| IBIS file stm32h523_533_lqfp64.ibs
[IBIS ver] 4.2
[File name] stm32h523_533_lqfp64.ibs
[File Rev] 0.2
[Date] 07-05-2024
[Source] Data Created at STMicroelectronics
[Notes]  File originated from ELDO simulations.
[Disclaimer]  This information is for modeling purpose only and is
   not guaranteed. The information is subject to change without
   notice.
[Copyright] Copyright 2024 STMicroelectronics Inc.
|   Component stm32h523_533_lqfp64
[Component] stm32h523_533_lqfp64
[Manufacturer] STMicroelectronics
[Package]
| variable   typ   min   max
R_pkg  0  NA  NA
L_pkg  0  NA  NA
C_pkg  0  NA  NA
[Pin]   signal_name   model_name
1  VBAT  power
2  PC13  io8_ft_i3c_spi_v33
3  PC14-OSC32_IN  io_ft_tamp
4  PC15-OSC32_OUT  io_ft_tamp
5  PH0-OSC_IN  io8_ft_i3c_spi
6  PH1-OSC_OUT  io8_ft_i3c_spi
7  NRST  ioreset_ft_v33
8  PC0  io8_ft_spi
9  PC1  io8_ft_spi
10  PC2  io8_ft_spi
11  PC3  io8_ft_spi
12  VSSA  nc
13  VDDA  nc
14  PA0  io8_ft_spi
15  PA1  io8_ft_spi_tamp
16  PA2  io8_ft_spi
17  PA3  io8_ft_spi
18  VSS  gnd
19  VDD  power
20  PA4  io8_ft_spi
21  PA5  io8_ft_spi
22  PA6  io8_ft_spi
23  PA7  io8_ft_spi
24  PC4  io8_ft_spi
25  PC5  io8_ft_spi
26  PB0  io8_ft_spi
27  PB1  io8_ft_spi
28  PB2  io8_ft_i3c_spi
29  PB10  io8_ft_i3c_spi
30  VCAP  nc
31  VSS  gnd
32  VDD  power
33  PB12  io8_ft_i3c_spi
34  PB13  nc
35  PB14  nc
36  PB15  io8_ft_spi
37  PC6  io8_ft_i3c_spi
38  PC7  io8_ft_i3c_spi
39  PC8  io8_ft_i3c_spi
40  PC9  io8_ft_i3c_spi
41  PA8  io8_ft_i3c_spi
42  PA9  io8_ft_i3c_spi
43  PA10  io8_ft_i3c_spi
44  PA11  io8usb_ft_i3c_spi_phy
45  PA12  io8usb_ft_i3c_spi_phy
46  PA13  io8_ft_i3c_spi
47  VSS  gnd
48  VDD  power
49  PA14  io8_ft_i3c_spi
50  PA15  io8_ft_i3c_spi
51  PC10  io8_ft_i3c_spi
52  PC11  io8_ft_i3c_spi
53  PC12  io8_ft_i3c_spi
54  PD2  io8_ft_i3c_spi
55  PB3  io8_ft_i3c_spi
56  PB4  io8_ft_i3c_spi
57  PB5  io8_ft_i3c_spi
58  PB6  io8_ft_i3c_spi
59  PB7  io8_ft_i3c_spi
60  BOOT0  vpphv
61  PB8  io8_ft_i3c_spi
62  VCAP  nc
63  VSS  gnd
64  VDD  power
[Package Model]   478-lqfp-7x7-64-240319
[Pin Mapping]   pulldown_ref   pullup_ref   | Comment
1  nc  vsw
2  gndio  vddio  | Depending on IO usage
| 2  gndio  vsw  | Depending on IO usage
3  gndio  vddio  | Depending on IO usage
| 3  gndio  vsw  | Depending on IO usage
4  gndio  vddio  | Depending on IO usage
| 4  gndio  vsw  | Depending on IO usage
5  gndio  vddio
6  gndio  vddio
7  gndio  vddio
8  gndio  vddio
9  gndio  vddio
10  gndio  vddio
11  gndio  vddio
12  nc  nc
13  nc  nc
14  gndio  vddio
15  gndio  vddio
16  gndio  vddio
17  gndio  vddio
18  gndio  nc
19  nc  vddio
20  gndio  vddio
21  gndio  vddio
22  gndio  vddio
23  gndio  vddio
24  gndio  vddio
25  gndio  vddio
26  gndio  vddio
27  gndio  vddio
28  gndio  vddio
29  gndio  vddio
30  nc  nc
31  gndio  nc
32  nc  vddio
33  gndio  vddio
34  nc  nc
35  nc  nc
36  gndio  vddio
37  gndio  vddio
38  gndio  vddio
39  gndio  vddio
40  gndio  vddio
41  gndio  vddio
42  gndio  vddio
43  gndio  vddio
44  gndio  vddio
45  gndio  vddio
46  gndio  vddio
47  gndio  nc
48  nc  vddio
49  gndio  vddio
50  gndio  vddio
51  gndio  vddio
52  gndio  vddio
53  gndio  vddio
54  gndio  vddio
55  gndio  vddio
56  gndio  vddio
57  gndio  vddio
58  gndio  vddio
59  gndio  vddio
60  gndio  vddio
61  gndio  vddio
62  nc  nc
63  gndio  nc
64  nc  vddio
|[Diff Pin]  inv_pin  vdiff  tdelay_typ  tdelay_min  tdelay_max
|45  44  NA  NA  NA  NA
[Model Selector] io8_ft_i3c_spi
io8_ft_spi_ls_1v2 "GPIO SPI - 5V tolerant - low speed - 1.2V range"
io8_ft_spi_ls_1v8 "GPIO SPI - 5V tolerant - low speed - 1.8V range"
io8_ft_spi_ls_3v3 "GPIO SPI - 5V tolerant - low speed - 3.3V range"
io8_ft_spi_ms_1v2 "GPIO SPI - 5V tolerant - med speed - 1.2V range"
io8_ft_spi_ms_1v8 "GPIO SPI - 5V tolerant - med speed - 1.8V range"
io8_ft_spi_ms_3v3 "GPIO SPI - 5V tolerant - med speed - 3.3V range"
io8_ft_spi_fs_1v2 "GPIO SPI - 5V tolerant - fast speed - 1.2V range"
io8_ft_spi_fs_1v8 "GPIO SPI - 5V tolerant - fast speed - 1.8V range"
io8_ft_spi_fs_3v3 "GPIO SPI - 5V tolerant - fast speed - 3.3V range"
io8_ft_spi_hs_1v2 "GPIO SPI - 5V tolerant - high speed - 1.2V range"
io8_ft_spi_hs_1v8 "GPIO SPI - 5V tolerant - high speed - 1.8V range"
io8_ft_spi_hs_3v3 "GPIO SPI - 5V tolerant - high speed - 3.3V range"
io8_ft_hslv_spi_ls_1v2 "GPIO SPI low volt opt - 5V tolerant - low speed - 1.2V range"
io8_ft_hslv_spi_ls_1v8 "GPIO SPI low volt opt - 5V tolerant - low speed - 1.8V range"
io8_ft_hslv_spi_ls_2v5 "GPIO SPI low volt opt - 5V tolerant - low speed - 2.5V range"
io8_ft_hslv_spi_ms_1v2 "GPIO SPI low volt opt - 5V tolerant - med speed - 1.2V range"
io8_ft_hslv_spi_ms_1v8 "GPIO SPI low volt opt - 5V tolerant - med speed - 1.8V range"
io8_ft_hslv_spi_ms_2v5 "GPIO SPI low volt opt - 5V tolerant - med speed - 2.5V range"
io8_ft_hslv_spi_fs_1v2 "GPIO SPI low volt opt - 5V tolerant - fast speed - 1.2V range"
io8_ft_hslv_spi_fs_1v8 "GPIO SPI low volt opt - 5V tolerant - fast speed - 1.8V range"
io8_ft_hslv_spi_fs_2v5 "GPIO SPI low volt opt - 5V tolerant - fast speed - 2.5V range"
io8_ft_hslv_spi_hs_1v2 "GPIO SPI low volt opt - 5V tolerant - high speed - 1.2V range"
io8_ft_hslv_spi_hs_1v8 "GPIO SPI low volt opt - 5V tolerant - high speed - 1.8V range"
io8_ft_hslv_spi_hs_2v5 "GPIO SPI low volt opt - 5V tolerant - high speed - 2.5V range"
io8_ft_i3c_spi_ls_1v2 "GPIO SPI with I3C open-drain - 5V tolerant - low speed - 1.2V range"
io8_ft_i3c_spi_ls_1v8 "GPIO SPI with I3C open-drain - 5V tolerant - low speed - 1.8V range"
io8_ft_i3c_spi_ls_3v3 "GPIO SPI with I3C open-drain - 5V tolerant - low speed - 3.3V range"
io8_ft_i3c_spi_ms_1v2 "GPIO SPI with I3C open-drain - 5V tolerant - med speed - 1.2V range"
io8_ft_i3c_spi_ms_1v8 "GPIO SPI with I3C open-drain - 5V tolerant - med speed - 1.8V range"
io8_ft_i3c_spi_ms_3v3 "GPIO SPI with I3C open-drain - 5V tolerant - med speed - 3.3V range"
io8_ft_i3c_spi_fs_1v2 "GPIO SPI with I3C open-drain - 5V tolerant - fast speed - 1.2V range"
io8_ft_i3c_spi_fs_1v8 "GPIO SPI with I3C open-drain - 5V tolerant - fast speed - 1.8V range"
io8_ft_i3c_spi_fs_3v3 "GPIO SPI with I3C open-drain - 5V tolerant - fast speed - 3.3V range"
io8_ft_i3c_spi_hs_1v2 "GPIO SPI with I3C open-drain - 5V tolerant - high speed - 1.2V range"
io8_ft_i3c_spi_hs_1v8 "GPIO SPI with I3C open-drain - 5V tolerant - high speed - 1.8V range"
io8_ft_i3c_spi_hs_3v3 "GPIO SPI with I3C open-drain - 5V tolerant - high speed - 3.3V range"
io8_ft_hslv_i3c_spi_ls_1v2 "GPIO SPI low volt opt with I3C open-drain - 5V tolerant - low speed - 1.2V range"
io8_ft_hslv_i3c_spi_ls_1v8 "GPIO SPI low volt opt with I3C open-drain - 5V tolerant - low speed - 1.8V range"
io8_ft_hslv_i3c_spi_ls_2v5 "GPIO SPI low volt opt with I3C open-drain - 5V tolerant - low speed - 2.5V range"
io8_ft_hslv_i3c_spi_ms_1v2 "GPIO SPI low volt opt with I3C open-drain - 5V tolerant - med speed - 1.2V range"
io8_ft_hslv_i3c_spi_ms_1v8 "GPIO SPI low volt opt with I3C open-drain - 5V tolerant - med speed - 1.8V range"
io8_ft_hslv_i3c_spi_ms_2v5 "GPIO SPI low volt opt with I3C open-drain - 5V tolerant - med speed - 2.5V range"
io8_ft_hslv_i3c_spi_fs_1v2 "GPIO SPI low volt opt with I3C open-drain - 5V tolerant - fast speed - 1.2V range"
io8_ft_hslv_i3c_spi_fs_1v8 "GPIO SPI low volt opt with I3C open-drain - 5V tolerant - fast speed - 1.8V range"
io8_ft_hslv_i3c_spi_fs_2v5 "GPIO SPI low volt opt with I3C open-drain - 5V tolerant - fast speed - 2.5V range"
io8_ft_hslv_i3c_spi_hs_1v2 "GPIO SPI low volt opt with I3C open-drain - 5V tolerant - high speed - 1.2V range"
io8_ft_hslv_i3c_spi_hs_1v8 "GPIO SPI low volt opt with I3C open-drain - 5V tolerant - high speed - 1.8V range"
io8_ft_hslv_i3c_spi_hs_2v5 "GPIO SPI low volt opt with I3C open-drain - 5V tolerant - high speed - 2.5V range"
io8_ft_i3c_fmp_spi_3v3 "GPIO SPI with I3C fm+ open-drain - 5V tolerant - 3.3V range"
io8_ft_i3c_fmp_spi_1v8 "GPIO SPI with I3C fm+ open-drain - 5V tolerant - 1.8V range"
io8_ft_i3c_fmp_spi_1v2 "GPIO SPI with I3C fm+ open-drain - 5V tolerant - 1.2V range"
[Model Selector] io8_ft_i3c_spi_v33
io8_ft_spi_v33_ls_1v2 ""GPIO SPI V33 - 5V tolerant - low speed - 1.2V range"
io8_ft_spi_v33_ls_1v8 ""GPIO SPI V33 - 5V tolerant - low speed - 1.8V range"
io8_ft_spi_v33_ls_3v3 ""GPIO SPI V33 - 5V tolerant - low speed - 3.3V range"
io8_ft_spi_v33_ms_1v2 ""GPIO SPI V33 - 5V tolerant - med speed - 1.2V range"
io8_ft_spi_v33_ms_1v8 ""GPIO SPI V33 - 5V tolerant - med speed - 1.8V range"
io8_ft_spi_v33_ms_3v3 ""GPIO SPI V33 - 5V tolerant - med speed - 3.3V range"
io8_ft_spi_v33_fs_1v2 ""GPIO SPI V33 - 5V tolerant - fast speed - 1.2V range
io8_ft_spi_v33_fs_1v8 ""GPIO SPI V33 - 5V tolerant - fast speed - 1.8V range
io8_ft_spi_v33_fs_3v3 ""GPIO SPI V33 - 5V tolerant - fast speed - 3.3V range
io8_ft_spi_v33_hs_1v2 ""GPIO SPI V33 - 5V tolerant - high speed - 1.2V range
io8_ft_spi_v33_hs_1v8 ""GPIO SPI V33 - 5V tolerant - high speed - 1.8V range
io8_ft_spi_v33_hs_3v3 ""GPIO SPI V33 - 5V tolerant - high speed - 3.3V range
io8_ft_hslv_spi_v33_ls_1v2 "GPIO SPI V33 low volt opt - 5V tolerant - low speed - 1.2V range""
io8_ft_hslv_spi_v33_ls_1v8 "GPIO SPI V33 low volt opt - 5V tolerant - low speed - 1.8V range""
io8_ft_hslv_spi_v33_ls_2v5 "GPIO SPI V33 low volt opt - 5V tolerant - low speed - 2.5V range""
io8_ft_hslv_spi_v33_ms_1v2 "GPIO SPI V33 low volt opt - 5V tolerant - med speed - 1.2V range""
io8_ft_hslv_spi_v33_ms_1v8 "GPIO SPI V33 low volt opt - 5V tolerant - med speed - 1.8V range""
io8_ft_hslv_spi_v33_ms_2v5 "GPIO SPI V33 low volt opt - 5V tolerant - med speed - 2.5V range""
io8_ft_hslv_spi_v33_fs_1v2 "GPIO SPI V33 low volt opt - 5V tolerant - fast speed - 1.2V range"
io8_ft_hslv_spi_v33_fs_1v8 "GPIO SPI V33 low volt opt - 5V tolerant - fast speed - 1.8V range"
io8_ft_hslv_spi_v33_fs_2v5 "GPIO SPI V33 low volt opt - 5V tolerant - fast speed - 2.5V range"
io8_ft_hslv_spi_v33_hs_1v2 "GPIO SPI V33 low volt opt - 5V tolerant - high speed - 1.2V range"
io8_ft_hslv_spi_v33_hs_1v8 "GPIO SPI V33 low volt opt - 5V tolerant - high speed - 1.8V range"
io8_ft_hslv_spi_v33_hs_2v5 "GPIO SPI V33 low volt opt - 5V tolerant - high speed - 2.5V range"
io8_ft_i3c_spi_v33_ls_1v2 "GPIO SPI V33 with I3C open-drain - 5V tolerant - low speed - 1.2V range"
io8_ft_i3c_spi_v33_ls_1v8 "GPIO SPI V33 with I3C open-drain - 5V tolerant - low speed - 1.8V range"
io8_ft_i3c_spi_v33_ls_3v3 "GPIO SPI V33 with I3C open-drain - 5V tolerant - low speed - 3.3V range"
io8_ft_i3c_spi_v33_ms_1v2 "GPIO SPI V33 with I3C open-drain - 5V tolerant - med speed - 1.2V range"
io8_ft_i3c_spi_v33_ms_1v8 "GPIO SPI V33 with I3C open-drain - 5V tolerant - med speed - 1.8V range"
io8_ft_i3c_spi_v33_ms_3v3 "GPIO SPI V33 with I3C open-drain - 5V tolerant - med speed - 3.3V range"
io8_ft_i3c_spi_v33_fs_1v2 "GPIO SPI V33 with I3C open-drain - 5V tolerant - fast speed - 1.2V range"
io8_ft_i3c_spi_v33_fs_1v8 "GPIO SPI V33 with I3C open-drain - 5V tolerant - fast speed - 1.8V range"
io8_ft_i3c_spi_v33_fs_3v3 "GPIO SPI V33 with I3C open-drain - 5V tolerant - fast speed - 3.3V range"
io8_ft_i3c_spi_v33_hs_1v2 "GPIO SPI V33 with I3C open-drain - 5V tolerant - high speed - 1.2V range"
io8_ft_i3c_spi_v33_hs_1v8 "GPIO SPI V33 with I3C open-drain - 5V tolerant - high speed - 1.8V range"
io8_ft_i3c_spi_v33_hs_3v3 "GPIO SPI V33 with I3C open-drain - 5V tolerant - high speed - 3.3V range"
io8_ft_hslv_i3c_spi_v33_ls_1v2 "GPIO SPI V33 low volt opt with I3C open-drain - 5V tolerant - low speed - 1.2V range"
io8_ft_hslv_i3c_spi_v33_ls_1v8 "GPIO SPI V33 low volt opt with I3C open-drain - 5V tolerant - low speed - 1.8V range"
io8_ft_hslv_i3c_spi_v33_ls_2v5 "GPIO SPI V33 low volt opt with I3C open-drain - 5V tolerant - low speed - 2.5V range"
io8_ft_hslv_i3c_spi_v33_ms_1v2 "GPIO SPI V33 low volt opt with I3C open-drain - 5V tolerant - med speed - 1.2V range"
io8_ft_hslv_i3c_spi_v33_ms_1v8 "GPIO SPI V33 low volt opt with I3C open-drain - 5V tolerant - med speed - 1.8V range"
io8_ft_hslv_i3c_spi_v33_ms_2v5 "GPIO SPI V33 low volt opt with I3C open-drain - 5V tolerant - med speed - 2.5V range"
io8_ft_hslv_i3c_spi_v33_fs_1v2 "GPIO SPI V33 low volt opt with I3C open-drain - 5V tolerant - fast speed - 1.2V range"
io8_ft_hslv_i3c_spi_v33_fs_1v8 "GPIO SPI V33 low volt opt with I3C open-drain - 5V tolerant - fast speed - 1.8V range"
io8_ft_hslv_i3c_spi_v33_fs_2v5 "GPIO SPI V33 low volt opt with I3C open-drain - 5V tolerant - fast speed - 2.5V range"
io8_ft_hslv_i3c_spi_v33_hs_1v2 "GPIO SPI V33 low volt opt with I3C open-drain - 5V tolerant - high speed - 1.2V range"
io8_ft_hslv_i3c_spi_v33_hs_1v8 "GPIO SPI V33 low volt opt with I3C open-drain - 5V tolerant - high speed - 1.8V range"
io8_ft_hslv_i3c_spi_v33_hs_2v5 "GPIO SPI V33 low volt opt with I3C open-drain - 5V tolerant - high speed - 2.5V range"
io8_ft_i3c_fmp_spi_v33_3v3 "GPIO SPI V33 with I3C fm+ open-drain - 5V tolerant - 3.3V range"
io8_ft_i3c_fmp_spi_v33_1v8 "GPIO SPI V33 with I3C fm+ open-drain - 5V tolerant - 1.8V range"
io8_ft_i3c_fmp_spi_v33_1v2 "GPIO SPI V33 with I3C fm+ open-drain - 5V tolerant - 1.2V range"
[Model Selector] io8_ft_spi
io8_ft_spi_ls_1v2 "GPIO SPI - 5V tolerant - low speed - 1.2V range"
io8_ft_spi_ls_1v8 "GPIO SPI - 5V tolerant - low speed - 1.8V range"
io8_ft_spi_ls_3v3 "GPIO SPI - 5V tolerant - low speed - 3.3V range"
io8_ft_spi_ms_1v2 "GPIO SPI- 5V tolerant - med speed - 1.2V range"
io8_ft_spi_ms_1v8 "GPIO SPI- 5V tolerant - med speed - 1.8V range"
io8_ft_spi_ms_3v3 "GPIO SPI- 5V tolerant - med speed - 3.3V range"
io8_ft_spi_fs_1v2 "GPIO SPI- 5V tolerant - fast speed - 1.2V range"
io8_ft_spi_fs_1v8 "GPIO SPI- 5V tolerant - fast speed - 1.8V range"
io8_ft_spi_fs_3v3 "GPIO SPI- 5V tolerant - fast speed - 3.3V range"
io8_ft_spi_hs_1v2 "GPIO SPI- 5V tolerant - high speed - 1.2V range"
io8_ft_spi_hs_1v8 "GPIO SPI- 5V tolerant - high speed - 1.8V range"
io8_ft_spi_hs_3v3 "GPIO SPI- 5V tolerant - high speed - 3.3V range"
io8_ft_hslv_spi_ls_1v2 "GPIO SPI low volt opt - 5V tolerant - low speed - 1.2V range"
io8_ft_hslv_spi_ls_1v8 "GPIO SPI low volt opt - 5V tolerant - low speed - 1.8V range"
io8_ft_hslv_spi_ls_2v5 "GPIO SPI low volt opt - 5V tolerant - low speed - 2.5V range"
io8_ft_hslv_spi_ms_1v2 "GPIO SPI low volt opt - 5V tolerant - med speed - 1.2V range"
io8_ft_hslv_spi_ms_1v8 "GPIO SPI low volt opt - 5V tolerant - med speed - 1.8V range"
io8_ft_hslv_spi_ms_2v5 "GPIO SPI low volt opt - 5V tolerant - med speed - 2.5V range"
io8_ft_hslv_spi_fs_1v2 "GPIO SPI low volt opt - 5V tolerant - fast speed - 1.2V range"
io8_ft_hslv_spi_fs_1v8 "GPIO SPI low volt opt - 5V tolerant - fast speed - 1.8V range"
io8_ft_hslv_spi_fs_2v5 "GPIO SPI low volt opt - 5V tolerant - fast speed - 2.5V range"
io8_ft_hslv_spi_hs_1v2 "GPIO SPI low volt opt - 5V tolerant - high speed - 1.2V range"
io8_ft_hslv_spi_hs_1v8 "GPIO SPI low volt opt - 5V tolerant - high speed - 1.8V range"
io8_ft_hslv_spi_hs_2v5 "GPIO SPI low volt opt - 5V tolerant - high speed - 2.5V range"
[Model Selector] io8_ft_spi_tamp
io8_ft_spi_ls_1v2 "GPIO SPI - 5V tolerant - low speed - 1.2V range"
io8_ft_spi_ls_1v8 "GPIO SPI - 5V tolerant - low speed - 1.8V range"
io8_ft_spi_ls_3v3 "GPIO SPI- 5V tolerant - low speed - 3.3V range"
io8_ft_spi_ms_1v2 "GPIO SPI - 5V tolerant - med speed - 1.2V range"
io8_ft_spi_ms_1v8 "GPIO SPI - 5V tolerant - med speed - 1.8V range"
io8_ft_spi_ms_3v3 "GPIO SPI - 5V tolerant - med speed - 3.3V range"
io8_ft_spi_fs_1v2 "GPIO SPI - 5V tolerant - fast speed - 1.2V range"
io8_ft_spi_fs_1v8 "GPIO SPI - 5V tolerant - fast speed - 1.8V range"
io8_ft_spi_fs_3v3 "GPIO SPI - 5V tolerant - fast speed - 3.3V range"
io8_ft_spi_hs_1v2 "GPIO SPI - 5V tolerant - high speed - 1.2V range"
io8_ft_spi_hs_1v8 "GPIO SPI - 5V tolerant - high speed - 1.8V range"
io8_ft_spi_hs_3v3 "GPIO SPI - 5V tolerant - high speed - 3.3V range"
io8_ft_hslv_spi_ls_1v2 "GPIO SPI low volt opt - 5V tolerant - low speed - 1.2V range"
io8_ft_hslv_spi_ls_1v8 "GPIO SPI low volt opt - 5V tolerant - low speed - 1.8V range"
io8_ft_hslv_spi_ls_2v5 "GPIO SPI low volt opt - 5V tolerant - low speed - 2.5V range"
io8_ft_hslv_spi_ms_1v2 "GPIO SPI low volt opt - 5V tolerant - med speed - 1.2V range"
io8_ft_hslv_spi_ms_1v8 "GPIO SPI low volt opt - 5V tolerant - med speed - 1.8V range"
io8_ft_hslv_spi_ms_2v5 "GPIO SPI low volt opt - 5V tolerant - med speed - 2.5V range"
io8_ft_hslv_spi_fs_1v2 "GPIO SPI low volt opt - 5V tolerant - fast speed - 1.2V range"
io8_ft_hslv_spi_fs_1v8 "GPIO SPI low volt opt - 5V tolerant - fast speed - 1.8V range"
io8_ft_hslv_spi_fs_2v5 "GPIO SPI low volt opt - 5V tolerant - fast speed - 2.5V range"
io8_ft_hslv_spi_hs_1v2 "GPIO SPI low volt opt - 5V tolerant - high speed - 1.2V range"
io8_ft_hslv_spi_hs_1v8 "GPIO SPI low volt opt - 5V tolerant - high speed - 1.8V range"
io8_ft_hslv_spi_hs_2v5 "GPIO SPI low volt opt - 5V tolerant - high speed - 2.5V range
io8_ft_tamp_v33_1v2 "IO tamper - 5V tolerant - 1.2V range"
io8_ft_tamp_v33_1v8 "IO tamper - 5V tolerant - 1.8V range"
io8_ft_tamp_v33_3v3 "IO tamper - 5V tolerant - 3.3V range"
[Model Selector] io8usb_ft_i3c_spi_phy
io8_ft_spi_ls_1v2 "GPIO SPI - 5V tolerant - low speed - 1.2V range"
io8_ft_spi_ls_1v8 "GPIO SPI - 5V tolerant - low speed - 1.8V range"
io8_ft_spi_ls_3v3 "GPIO SPI - 5V tolerant - low speed - 3.3V range"
io8_ft_spi_ms_1v2 "GPIO SPI - 5V tolerant - med speed - 1.2V range"
io8_ft_spi_ms_1v8 "GPIO SPI - 5V tolerant - med speed - 1.8V range"
io8_ft_spi_ms_3v3 "GPIO SPI - 5V tolerant - med speed - 3.3V range"
io8_ft_spi_fs_1v2 "GPIO SPI - 5V tolerant - fast speed - 1.2V range"
io8_ft_spi_fs_1v8 "GPIO SPI - 5V tolerant - fast speed - 1.8V range"
io8_ft_spi_fs_3v3 "GPIO SPI - 5V tolerant - fast speed - 3.3V range"
io8_ft_spi_hs_1v2 "GPIO SPI - 5V tolerant - high speed - 1.2V range"
io8_ft_spi_hs_1v8 "GPIO SPI - 5V tolerant - high speed - 1.8V range"
io8_ft_spi_hs_3v3 "GPIO SPI - 5V tolerant - high speed - 3.3V range"
io8_ft_hslv_spi_ls_1v2 "GPIO SPI low volt opt - 5V tolerant - low speed - 1.2V range"
io8_ft_hslv_spi_ls_1v8 "GPIO SPI low volt opt - 5V tolerant - low speed - 1.8V range"
io8_ft_hslv_spi_ls_2v5 "GPIO SPI low volt opt - 5V tolerant - low speed - 2.5V range"
io8_ft_hslv_spi_ms_1v2 "GPIO SPI low volt opt - 5V tolerant - med speed - 1.2V range"
io8_ft_hslv_spi_ms_1v8 "GPIO SPI low volt opt - 5V tolerant - med speed - 1.8V range"
io8_ft_hslv_spi_ms_2v5 "GPIO SPI low volt opt - 5V tolerant - med speed - 2.5V range"
io8_ft_hslv_spi_fs_1v2 "GPIO SPI low volt opt - 5V tolerant - fast speed - 1.2V range"
io8_ft_hslv_spi_fs_1v8 "GPIO SPI low volt opt - 5V tolerant - fast speed - 1.8V range"
io8_ft_hslv_spi_fs_2v5 "GPIO SPI low volt opt - 5V tolerant - fast speed - 2.5V range"
io8_ft_hslv_spi_hs_1v2 "GPIO SPI low volt opt - 5V tolerant - high speed - 1.2V range"
io8_ft_hslv_spi_hs_1v8 "GPIO SPI low volt opt - 5V tolerant - high speed - 1.8V range"
io8_ft_hslv_spi_hs_2v5 "GPIO SPI low volt opt - 5V tolerant - high speed - 2.5V range"
io8_ft_i3c_spi_ls_1v2 "GPIO SPI  with I3C open-drain - 5V tolerant - low speed - 1.2V range"
io8_ft_i3c_spi_ls_1v8 "GPIO SPI  with I3C open-drain - 5V tolerant - low speed - 1.8V range"
io8_ft_i3c_spi_ls_3v3 "GPIO SPI  with I3C open-drain - 5V tolerant - low speed - 3.3V range"
io8_ft_i3c_spi_ms_1v2 "GPIO SPI  with I3C open-drain - 5V tolerant - med speed - 1.2V range"
io8_ft_i3c_spi_ms_1v8 "GPIO SPI  with I3C open-drain - 5V tolerant - med speed - 1.8V range"
io8_ft_i3c_spi_ms_3v3 "GPIO SPI  with I3C open-drain - 5V tolerant - med speed - 3.3V range"
io8_ft_i3c_spi_fs_1v2 "GPIO SPI  with I3C open-drain - 5V tolerant - fast speed - 1.2V range"
io8_ft_i3c_spi_fs_1v8 "GPIO SPI  with I3C open-drain - 5V tolerant - fast speed - 1.8V range"
io8_ft_i3c_spi_fs_3v3 "GPIO SPI  with I3C open-drain - 5V tolerant - fast speed - 3.3V range"
io8_ft_i3c_spi_hs_1v2 "GPIO SPI  with I3C open-drain - 5V tolerant - high speed - 1.2V range"
io8_ft_i3c_spi_hs_1v8 "GPIO SPI  with I3C open-drain - 5V tolerant - high speed - 1.8V range"
io8_ft_i3c_spi_hs_3v3 "GPIO SPI  with I3C open-drain - 5V tolerant - high speed - 3.3V range"
io8_ft_hslv_i3c_spi_ls_1v2 "GPIO SPI  low volt opt with I3C open-drain - 5V tolerant - low speed - 1.2V range"
io8_ft_hslv_i3c_spi_ls_1v8 "GPIO SPI  low volt opt with I3C open-drain - 5V tolerant - low speed - 1.8V range"
io8_ft_hslv_i3c_spi_ls_2v5 "GPIO SPI  low volt opt with I3C open-drain - 5V tolerant - low speed - 2.5V range"
io8_ft_hslv_i3c_spi_ms_1v2 "GPIO SPI  low volt opt with I3C open-drain - 5V tolerant - med speed - 1.2V range"
io8_ft_hslv_i3c_spi_ms_1v8 "GPIO SPI  low volt opt with I3C open-drain - 5V tolerant - med speed - 1.8V range"
io8_ft_hslv_i3c_spi_ms_2v5 "GPIO SPI  low volt opt with I3C open-drain - 5V tolerant - med speed - 2.5V range"
io8_ft_hslv_i3c_spi_fs_1v2 "GPIO SPI  low volt opt with I3C open-drain - 5V tolerant - fast speed - 1.2V range"
io8_ft_hslv_i3c_spi_fs_1v8 "GPIO SPI  low volt opt with I3C open-drain - 5V tolerant - fast speed - 1.8V range"
io8_ft_hslv_i3c_spi_fs_2v5 "GPIO SPI  low volt opt with I3C open-drain - 5V tolerant - fast speed - 2.5V range"
io8_ft_hslv_i3c_spi_hs_1v2 "GPIO SPI  low volt opt with I3C open-drain - 5V tolerant - high speed - 1.2V range"
io8_ft_hslv_i3c_spi_hs_1v8 "GPIO SPI  low volt opt with I3C open-drain - 5V tolerant - high speed - 1.8V range"
io8_ft_hslv_i3c_spi_hs_2v5 "GPIO SPI  low volt opt with I3C open-drain - 5V tolerant - high speed - 2.5V range"
io8_ft_i3c_fmp_spi_3v3 "GPIO SPI  with I3C fm+ open-drain - 5V tolerant - 3.3V range"
io8_ft_i3c_fmp_spi_1v8 "GPIO SPI  with I3C fm+ open-drain - 5V tolerant - 1.8V range"
io8_ft_i3c_fmp_spi_1v2 "GPIO SPI  with I3C fm+ open-drain - 5V tolerant - 1.2V range"
io8usb_ft_phy_ls_2v5 "USB PHY - 5V tolerant - low speed - 2.5V range"
io8usb_ft_phy_ls_3v3 "USB PHY - 5V tolerant - low speed - 3.3V range
io8usb_ft_phy_fs_2v5 "USB PHY - 5V tolerant - fast speed - 2.5V range"
io8usb_ft_phy_fs_3v3 "USB PHY - 5V tolerant - fast speed - 3.3V range"
[Model Selector] io_ft_tamp
io_ft_tamp_3v3 "IO tamper - 5V tolerant - 3.3V range"
io_ft_tamp_1v8 "IO tamper - 5V tolerant - 1.8V range"
io_ft_tamp_1v2 "IO tamper - 5V tolerant - 1.2V range"
[Model Selector] ioreset_ft_v33
ioreset_ft_v33_1v2 "Reset PAD. 5V tolerant. 1.2V range"
ioreset_ft_v33_1v8 "Reset PAD. 5V tolerant. 1.8V range"
ioreset_ft_v33_3v3 "Reset PAD. 5V tolerant. 3.3V range"
[Model Selector] vpphv
vpphv_1v2 "Flash Test cell v33 = 1.2 V range"
vpphv_1v8 "Flash Test cell v33 = 1.8 V range"
vpphv_3v3 "Flash Test cell v33 = 3.3 V range"
[Define Package Model]  478-lqfp-7x7-64-240319
[Manufacturer]  Unknown
[OEM]  Unknown
[Description]  None
[Number Of Pins]  61
[Pin Numbers]
| Pin Num   Terminal Name
7 | NRST
14 | PA0
15 | PA1
16 | PA2
17 | PA3
20 | PA4
21 | PA5
22 | PA6
23 | PA7
41 | PA8
42 | PA9
43 | PA10
44 | PA11
45 | PA12
46 | PA13
49 | PA14
50 | PA15
26 | PB0
27 | PB1
28 | PB2
55 | PB3
56 | PB4
57 | PB5
58 | PB6
59 | PB7
61 | PB8
29 | PB10
33 | PB12
34 | PB13
35 | PB14
36 | PB15
8 | PC0
9 | PC1
10 | PC2
11 | PC3
24 | PC4
25 | PC5
37 | PC6
38 | PC7
39 | PC8
40 | PC9
51 | PC10
52 | PC11
53 | PC12
2 | PC13
3 | PC14-OSC32_IN
4 | PC15-OSC32_OUT
54 | PD2
5 | PH0-OSC_IN
6 | PH1-OSC_OUT
1 | VBAT
30 | VCAP
62 | VCAP
32 | VDD
48 | VDD
19 | VDD
64 | VDD
13 | VDDA
60 | BOOT0
18 | VSS
12 | VSSA
|[Merged Pins]  18
|31  |  VSS
|47  |  VSS
|63  |  VSS
[Model Data]
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[End Model Data]
[End Package Model]
|End [Component]
| Models and submodels in the file (118): io8_ft_hslv_i3c_spi_fs_1v2 (I/O_open_drain), io8_ft_hslv_i3c_spi_fs_1v8 (I/O_open_drain), io8_ft_hslv_i3c_spi_fs_2v5 (I/O_open_drain), io8_ft_hslv_i3c_spi_hs_1v2 (I/O_open_drain), io8_ft_hslv_i3c_spi_hs_1v8 (I/O_open_drain), io8_ft_hslv_i3c_spi_hs_2v5 (I/O_open_drain), io8_ft_hslv_i3c_spi_ls_1v2 (I/O_open_drain), io8_ft_hslv_i3c_spi_ls_1v8 (I/O_open_drain), io8_ft_hslv_i3c_spi_ls_2v5 (I/O_open_drain), io8_ft_hslv_i3c_spi_ms_1v2 (I/O_open_drain), io8_ft_hslv_i3c_spi_ms_1v8 (I/O_open_drain), io8_ft_hslv_i3c_spi_ms_2v5 (I/O_open_drain), io8_ft_hslv_i3c_spi_v33_fs_1v2 (I/O_open_drain), io8_ft_hslv_i3c_spi_v33_fs_1v8 (I/O_open_drain), io8_ft_hslv_i3c_spi_v33_fs_2v5 (I/O_open_drain), io8_ft_hslv_i3c_spi_v33_hs_1v2 (I/O_open_drain), io8_ft_hslv_i3c_spi_v33_hs_1v8 (I/O_open_drain), io8_ft_hslv_i3c_spi_v33_hs_2v5 (I/O_open_drain), io8_ft_hslv_i3c_spi_v33_ls_1v2 (I/O_open_drain), io8_ft_hslv_i3c_spi_v33_ls_1v8 (I/O_open_drain), io8_ft_hslv_i3c_spi_v33_ls_2v5 (I/O_open_drain), io8_ft_hslv_i3c_spi_v33_ms_1v2 (I/O_open_drain), io8_ft_hslv_i3c_spi_v33_ms_1v8 (I/O_open_drain), io8_ft_hslv_i3c_spi_v33_ms_2v5 (I/O_open_drain), io8_ft_hslv_spi_fs_1v2 (I/O), io8_ft_hslv_spi_fs_1v8 (I/O), io8_ft_hslv_spi_fs_2v5 (I/O), io8_ft_hslv_spi_hs_1v2 (I/O), io8_ft_hslv_spi_hs_1v8 (I/O), io8_ft_hslv_spi_hs_2v5 (I/O), io8_ft_hslv_spi_ls_1v2 (I/O), io8_ft_hslv_spi_ls_1v8 (I/O), io8_ft_hslv_spi_ls_2v5 (I/O), io8_ft_hslv_spi_ms_1v2 (I/O), io8_ft_hslv_spi_ms_1v8 (I/O), io8_ft_hslv_spi_ms_2v5 (I/O), io8_ft_hslv_spi_v33_fs_1v2 (I/O), io8_ft_hslv_spi_v33_fs_1v8 (I/O), io8_ft_hslv_spi_v33_fs_2v5 (I/O), io8_ft_hslv_spi_v33_hs_1v2 (I/O), io8_ft_hslv_spi_v33_hs_1v8 (I/O), io8_ft_hslv_spi_v33_hs_2v5 (I/O), io8_ft_hslv_spi_v33_ls_1v2 (I/O), io8_ft_hslv_spi_v33_ls_1v8 (I/O), io8_ft_hslv_spi_v33_ls_2v5 (I/O), io8_ft_hslv_spi_v33_ms_1v2 (I/O), io8_ft_hslv_spi_v33_ms_1v8 (I/O), io8_ft_hslv_spi_v33_ms_2v5 (I/O), io8_ft_i3c_fmp_spi_1v2 (I/O_open_drain), io8_ft_i3c_fmp_spi_1v8 (I/O_open_drain), io8_ft_i3c_fmp_spi_3v3 (I/O_open_drain), io8_ft_i3c_fmp_spi_v33_1v2 (I/O_open_drain), io8_ft_i3c_fmp_spi_v33_1v8 (I/O_open_drain), io8_ft_i3c_fmp_spi_v33_3v3 (I/O_open_drain), io8_ft_i3c_spi_fs_1v2 (I/O_open_drain), io8_ft_i3c_spi_fs_1v8 (I/O_open_drain), io8_ft_i3c_spi_fs_3v3 (I/O_open_drain), io8_ft_i3c_spi_hs_1v2 (I/O_open_drain), io8_ft_i3c_spi_hs_1v8 (I/O_open_drain), io8_ft_i3c_spi_hs_3v3 (I/O_open_drain), io8_ft_i3c_spi_ls_1v2 (I/O_open_drain), io8_ft_i3c_spi_ls_1v8 (I/O_open_drain), io8_ft_i3c_spi_ls_3v3 (I/O_open_drain), io8_ft_i3c_spi_ms_1v2 (I/O_open_drain), io8_ft_i3c_spi_ms_1v8 (I/O_open_drain), io8_ft_i3c_spi_ms_3v3 (I/O_open_drain), io8_ft_i3c_spi_v33_fs_1v2 (I/O_open_drain), io8_ft_i3c_spi_v33_fs_1v8 (I/O_open_drain), io8_ft_i3c_spi_v33_fs_3v3 (I/O_open_drain), io8_ft_i3c_spi_v33_hs_1v2 (I/O_open_drain), io8_ft_i3c_spi_v33_hs_1v8 (I/O_open_drain), io8_ft_i3c_spi_v33_hs_3v3 (I/O_open_drain), io8_ft_i3c_spi_v33_ls_1v2 (I/O_open_drain), io8_ft_i3c_spi_v33_ls_1v8 (I/O_open_drain), io8_ft_i3c_spi_v33_ls_3v3 (I/O_open_drain), io8_ft_i3c_spi_v33_ms_1v2 (I/O_open_drain), io8_ft_i3c_spi_v33_ms_1v8 (I/O_open_drain), io8_ft_i3c_spi_v33_ms_3v3 (I/O_open_drain), io8_ft_spi_fs_1v2 (I/O), io8_ft_spi_fs_1v8 (I/O)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
